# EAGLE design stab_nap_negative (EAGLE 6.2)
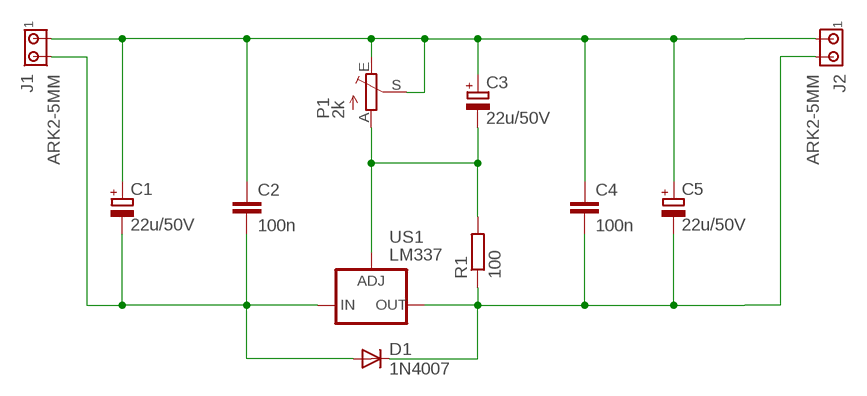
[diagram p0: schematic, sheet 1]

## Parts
C1  22u/50V  CPOL-EUE2.5-6  [E2,5-6]
C2  100n  C-EU050-025X075  [C050-025X075]
C3  22u/50V  CPOL-EUE2.5-6  [E2,5-6]
C4  100n  C-EU050-025X075  [C050-025X075]
C5  22u/50V  CPOL-EUE2.5-6  [E2,5-6]
D1  1N4007  1N4004  [DO41-10]
J1  ARK2-5MM  [2PIN-5MM]
J2  ARK2-5MM  [2PIN-5MM]
P1  2k  TRIM_EU-B64Y  [B64Y]
R1  100  R-EU_0207/7  [0207/7]
US1  LM337  LM337TS  [337TS]

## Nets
N$1: C1.+ C2.1 C3.+ C4.1 C5.+ J1.P$1 J2.P$1 P1.E P1.S
N$2: C1.- C2.2 D1.A J1.P$2 US1.2(IN)
N$11: C3.- P1.A R1.2 US1.1(ADJ)
N$12: C4.2 C5.- D1.C J2.P$2 R1.1 US1.3(OUT)

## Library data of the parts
C1 C3 C5 = rcl:CPOL-EU: POLARIZED CAPACITOR, European symbol
C2 C4 = rcl:C-EU: CAPACITOR, European symbol
D1 = diode:1N4004: DIODE
J1 J2 = zlacza_futrzak:ARK2: ARK 2
P1 = pot:TRIM_EU-: POTENTIOMETER
R1 = rcl:R-EU_: RESISTOR, European symbol
US1 = v-reg:LM337TS: VOLTAGE REGULATOR

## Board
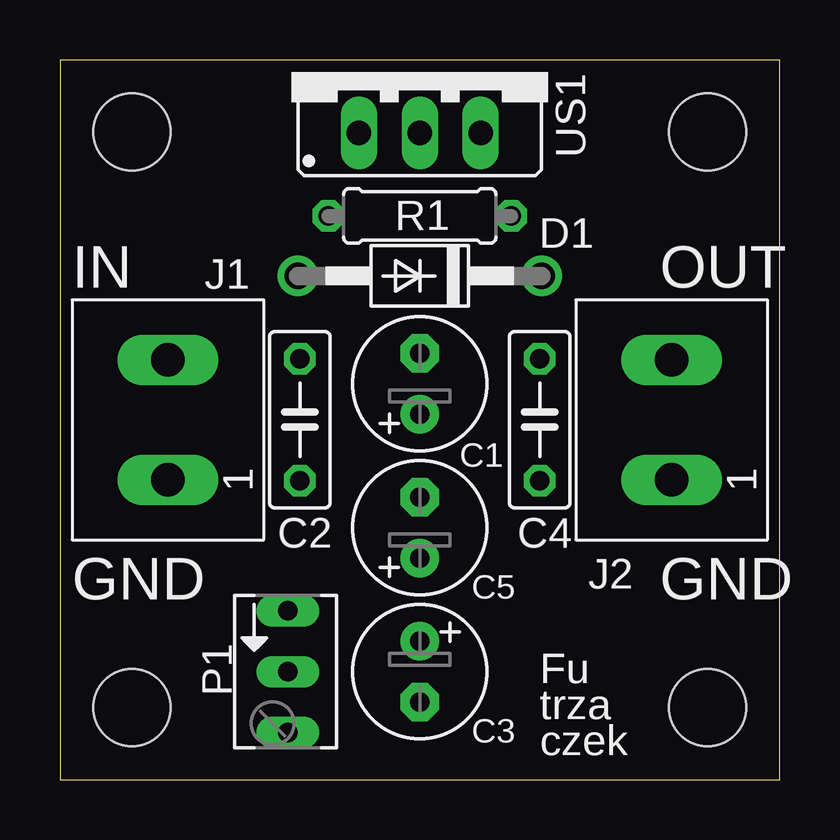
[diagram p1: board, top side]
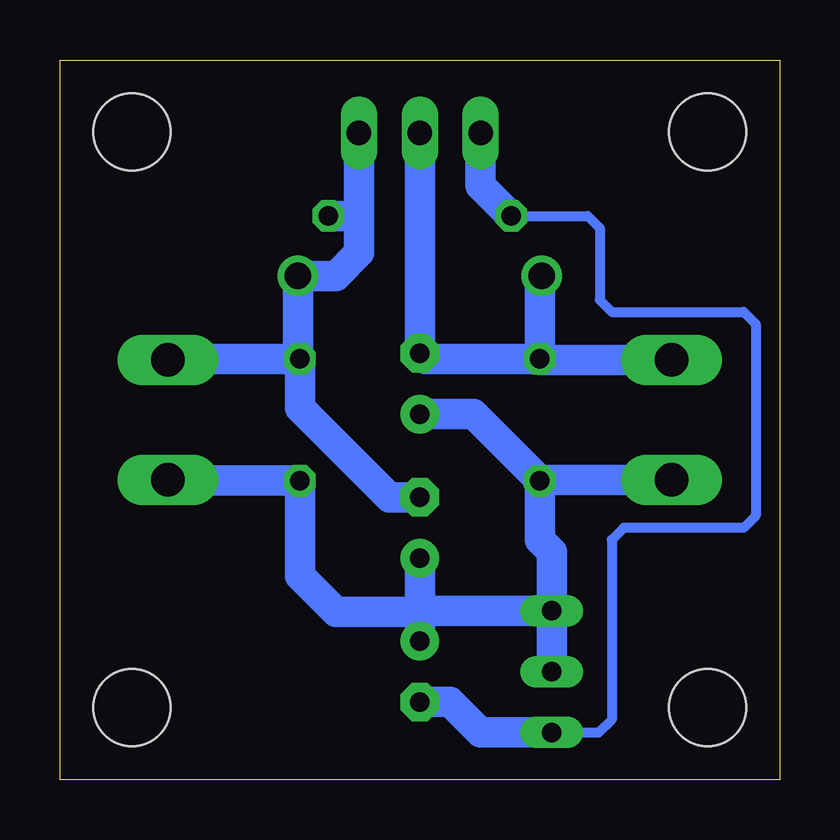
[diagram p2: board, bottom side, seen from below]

Size 30 x 30 mm. Coordinates in mm from the lower left corner, seen from the top.
Outline: 0,0 30,0 30,30 0,30 0,0
Copper layers (1*16): Top 0.035mm / dielectric 1.5mm / Bottom 0.035mm
Design rules: minimum track width 10mil, minimum drill 23mil, track to track 8mil, track to pad 8mil, pad to pad 8mil, via to via 8mil, smd to smd 8mil, copper to edge 20mil, drill to drill 8mil, minimum pad ring 10mil, minimum via ring 8mil, stop-mask expansion 4mil, vias tented up to drill 0mil, thermal gap 10mil
Holes 3.2 mm at 3,3 3,27 27,27 27,3

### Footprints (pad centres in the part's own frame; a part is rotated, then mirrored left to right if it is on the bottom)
E2,5-6 = drill 0.813 pad 1.6: + -1.27,0 | drill 0.813 pad 1.6 octagon: - 1.27,0
C050-025X075 = drill 0.813 octagon: 1 -2.54,0; 2 2.54,0
DO41-10 = drill 1.118: A 5.08,0; C -5.08,0
2PIN-5MM = drill 1.4 long: P$1 -2.5,0; P$2 2.5,0
B64Y = drill 0.813 long: A 2.54,0; E -2.54,0; S 0,0
0207/7 = drill 0.813 octagon: 1 -3.81,0; 2 3.81,0
337TS = drill 1.016 long: 1 -2.54,-2.54; 2 0,-2.54; 3 2.54,-2.54

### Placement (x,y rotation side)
C1  15,16.5 90 top
C2  10,15 90 top
C3  15,4.5 270 top
C4  20,15 90 top
C5  15,10.5 90 top
D1  15,21 180 top
J1  4.5,15 90 top
J2  25.5,15 90 top
P1  9.5,4.5 270 top
R1  15,23.5 180 top
US1  15,29.5 0 top

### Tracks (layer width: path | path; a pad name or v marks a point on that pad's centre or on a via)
N$1
  Bottom 1.27: J1.P$1 9.96,12.5 C2.1 | J2.P$1 25.46,12.46 C4.1 20,8.5 18.5,7 15,7 | P1.S P1.E | C3.+ 15,7 | 15,7 C5.+ | P1.E 14.96,7.04 15,7 | P1.E 9.5,9.5 10,10 C2.1 | C1.+ 12.77,15.23 C2.1
N$2
  Bottom 1.27: J1.P$2 9.96,17.5 C2.2 | C2.2 14.77,17.54 C1.- US1.2 | C2.2 10,20.92 D1.A
N$11
  Bottom 0.406: R1.2 8,23.5 7.5,23 7.5,20 7,19.5 1.5,19.5 1,19 1,11 1.5,10.5 6.5,10.5 7,10 7,2.5 7.54,1.96 P1.A
  Bottom 1.27: C3.- 13.73,3.23 13,2.5 12.46,1.96 P1.A | US1.1 12.46,24.77 R1.2
N$12
  Bottom 1.27: US1.3 17.54,23.5 | 17.54,23.5 17.54,21.96 18.5,21 D1.C 20.08,17.62 C4.2 | R1.1 17.54,23.5 | C4.2 25.46,17.54 J2.P$2 | C4.2 20,15.5 17.5,13 | 17.5,13 17,12.5 | C5.- 16.27,11.77 17.5,13

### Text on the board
tPlace: IN | OUT | GND | GND | Fu | trza | czek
